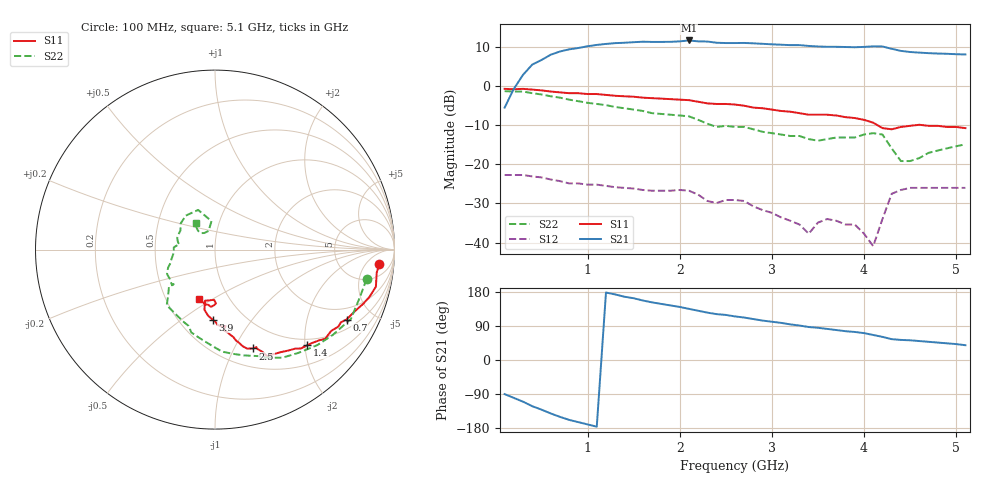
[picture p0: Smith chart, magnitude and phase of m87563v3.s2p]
!  MGA-87563 S PARAMETERS
!  Vd = 3 V  LAST UPDATED 12-21-94
# ghz s ma r 50
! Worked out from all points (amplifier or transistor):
!   51 points, 100 MHz to 5.1 GHz, reference 50 ohm
!   highest |S21| = 11.6 dB at 2.1 GHz (marker M1)
!   |S21| within 3 dB of that: 678.5 MHz to 4.531 GHz (3.853 GHz wide, 148 % of centre)
!   unconditionally stable (mu >= 1): 1.462 GHz to end of sweep
!   at 900 MHz: K = 0.65, MSG = 17.3 dB, |S12| = -24.9 dB
!   at 2.6 GHz: K = 2.45, MAG = 13.4 dB, |S12| = -29.1 dB
!   at 5.1 GHz: K = 3.52, MAG = 8.7 dB, |S12| = -26.0 dB
!   lowest NFmin = 1.51 dB at 2.5 GHz
!   S11 on the Smith chart (normalised r, x): 100 MHz: 11, -12; 700 MHz: 1.39, -3.49; 1.4 GHz: 0.87, -2.05; 2.5 GHz: 0.70, -1.19; 3.9 GHz: 0.72, -0.66; 5.1 GHz: 0.72, -0.44
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0.1  0.92 -5.0  0.53 -90.0  0.073 -7.0  0.86 -11.0
0.3  0.92 -13.0  1.39 -110.0  0.073 -12.0  0.85 -27.0
0.4  0.9 -17.0  1.88 -122.0  0.07 -18.0  0.81 -36.0
0.6  0.85 -24.0  2.51 -141.0  0.064 -23.0  0.74 -51.0
0.7  0.83 -28.0  2.76 -150.0  0.061 -25.0  0.71 -58.0
1  0.79 -35.0  3.22 -170.0  0.055 -26.0  0.61 -75.0
1.2  0.77 -41.0  3.45 178.0  0.053 -30.0  0.57 -86.0
1.4  0.74 -46.0  3.57 167.0  0.05 -32.0  0.52 -95.0
1.8  0.69 -55.0  3.66 148.0  0.046 -35.0  0.44 -113.0
2.1  0.66 -64.0  3.82 135.0  0.046 -48.0  0.41 -131.0
2.3  0.6 -67.0  3.7 125.0  0.034 -51.0  0.33 -141.0
2.5  0.59 -69.0  3.54 119.0  0.035 -40.0  0.31 -141.0
2.6  0.58 -72.0  3.54 115.0  0.035 -46.0  0.3 -147.0
2.9  0.52 -77.0  3.46 104.0  0.026 -52.0  0.26 -163.0
3.4  0.43 -82.0  3.25 87.0  0.013 -19.0  0.21 173.0
3.5  0.43 -83.0  3.2 85.0  0.018 -12.0  0.2 172.0
3.9  0.39 -92.0  3.13 74.0  0.017 -12.0  0.22 151.0
4.1  0.34 -100.0  3.21 66.0  0.009 24.0  0.25 131.0
4.2  0.29 -101.0  3.2 61.0  0.02 70.0  0.24 113.0
4.3  0.28 -91.0  2.99 55.0  0.042 50.0  0.16 97.0
4.5  0.31 -91.0  2.72 52.0  0.05 20.0  0.11 123.0
5.1  0.29 -108.0  2.53 39.0  0.05 -5.0  0.18 126.0
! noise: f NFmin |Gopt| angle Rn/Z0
0.1  3.48  0.74  -19  2.11
0.6  2.41  0.7  5  1.43
1.2  1.59  0.67  22  0.83
1.7  1.6  0.67  32  0.72
2.3  1.53  0.64  40  0.59
2.8  1.55  0.6  46  0.53
3.4  1.75  0.56  54  0.55
3.9  1.95  0.53  61  0.58
4.5  2.09  0.49  70  0.58
5.1  2.13  0.45  81  0.52
